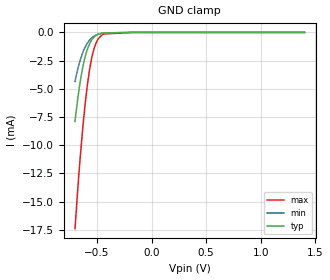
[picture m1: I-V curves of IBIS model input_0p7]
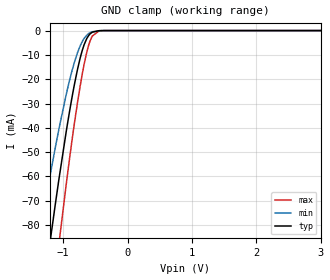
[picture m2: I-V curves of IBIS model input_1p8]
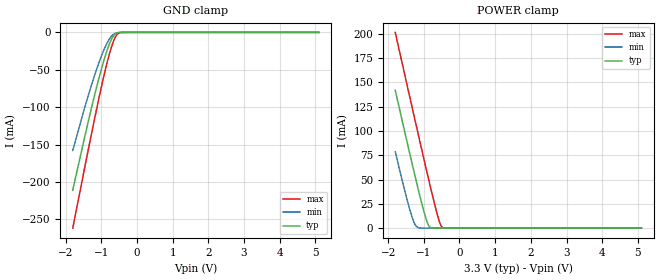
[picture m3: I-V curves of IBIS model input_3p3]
| Texas Instruments Incorporated
| SN74AXC4T774 4-Bit Dual-Supply Bus Transceiver with Independent Direction
| Control, Configurable Voltage Translation, and Tri-State Outputs
[IBIS Ver]   4.1
[File name]   sn74axc4t774.ibs
[Date]   04/15/2019
[File Rev]   1.0
[Source]
| Texas Instruments Incorporated.
| Analog-eLab Design Center, HPA
| 12500 TI Blvd
| Dallas, TX -75243
[Notes]   Revision History:
| Rev 1.0: 04/15/2019
| - Initial version of the model
| - Model generated from simulations in SPECTRE
| - C_comp although listed in numerical order of value are
|   obtained from varying PVT conditions. For PVT conditions for
|   each specific value refer the buffer description under
|   respective [Model]. IBIS model user is responsible for using
|   appropriate C_comp to simulate for Signal Integrity.
| - Warnings regarding combined Non-monotonicity of various models have been
|   reviewd and considered minor and can be ignored.
| - Model names with a trailing _0p7 contain the model for 0.7V operation.
|   Model names with a trailing _1p8 contain the model for 1.8V operation.
|   Model names with a trailing _3p3 contain the model for 3.3V operation.
[Disclaimer]
| This model is designed as an aid for customers of Texas Instruments.
| TI and its licensors and suppliers make no warranties, either expressed
| or implied, with respect to this  model, including the warranties of
| merchantability or fitness for a particular purpose. The model is
| provided solely on an "as is" basis. The entire risk as to its quality
| and performance is with the customer.
| This model is subject to change without notice. Texas Instruments
| Incorporated is not responsible for updating this model.
[Copyright]
(C) Copyright 2019 Texas Instruments Incorporated.All rights reserved.
|  Component SN74AXC4T774BQB 16-Pin VQFN - BQB package
|  Part # SN74AXC4T774BQB
[Component]   SN74AXC4T774BQB
[Manufacturer]  TI
[Package]   |16 VQFN - BQB package
|   typ   min   max
R_pkg   0.05   0.04   0.06
L_pkg   1.0nH   0.8nH   1.2nH
C_pkg   0.2pF   0.16pF   0.24pF
[Pin]  signal_name model_name   R_pin   L_pin   C_pin
1   DIR1   input   NA   NA   NA
2   DIR2   input   NA   NA   NA
3   A1   io   NA   NA   NA
4   A2   io   NA   NA   NA
5   A3   io   NA   NA   NA
6   A4   io   NA   NA   NA
7   DIR3   input   NA   NA   NA
8   DIR4   input   NA   NA   NA
9   nOE   input   NA   NA   NA
10   GND   gnd   NA   NA   NA
11   B4   io   NA   NA   NA
12   B3   io   NA   NA   NA
13   B2   io   NA   NA   NA
14   B1   io   NA   NA   NA
15   VCCB   power   NA   NA   NA
16   VCCA   power   NA   NA   NA
|  Component SN74AXC4T774PW 16-Pin TSSOP - PW package
|  Part # SN74AXC4T774PW
[Component]   SN74AXC4T774PW
[Manufacturer]  TI
[Package]   |16 TSSOP - PW package
|   typ   min   max
R_pkg   0.05   0.04   0.06
L_pkg   1.0nH   0.8nH   1.2nH
C_pkg   0.2pF   0.16pF   0.24pF
[Pin]  signal_name model_name   R_pin   L_pin   C_pin
1   DIR1   input   NA   NA   NA
2   DIR2   input   NA   NA   NA
3   A1   io   NA   NA   NA
4   A2   io   NA   NA   NA
5   A3   io   NA   NA   NA
6   A4   io   NA   NA   NA
7   DIR3   input   NA   NA   NA
8   DIR4   input   NA   NA   NA
9   nOE   input   NA   NA   NA
10   GND   gnd   NA   NA   NA
11   B4   io   NA   NA   NA
12   B3   io   NA   NA   NA
13   B2   io   NA   NA   NA
14   B1   io   NA   NA   NA
15   VCCB   power   NA   NA   NA
16   VCCA   power   NA   NA   NA
|  Component SN74AXC4T774RSV 16-Pin UQFN - RSV package
|  Part # SN74AXC4T774RSV
[Component]   SN74AXC4T774RSV
[Manufacturer]  TI
[Package]   |16 UQFN - RSV package
|   typ   min   max
R_pkg   0.05   0.04   0.06
L_pkg   1.0nH   0.8nH   1.2nH
C_pkg   0.2pF   0.16pF   0.24pF
[Pin]  signal_name model_name   R_pin   L_pin   C_pin
1   A1   io   NA   NA   NA
2   A2   io   NA   NA   NA
3   A3   io   NA   NA   NA
4   A4   io   NA   NA   NA
5   DIR3   input   NA   NA   NA
6   DIR4   input   NA   NA   NA
7   nOE   input   NA   NA   NA
8   GND   gnd   NA   NA   NA
9   B4   io   NA   NA   NA
10   B3   io   NA   NA   NA
11   B2   io   NA   NA   NA
12   B1   io   NA   NA   NA
13   VCCB   power   NA   NA   NA
14   VCCA   power   NA   NA   NA
15   DIR1   input   NA   NA   NA
16   DIR2   input   NA   NA   NA
|   Model Selectors
[Model Selector] input
input_0p7   0.7V   digital Input
input_1p8   1.8V   digital Input
input_3p3   3.3V   digital Input
[Model Selector] io
io_0p7_x   0.7V   digital I/O   |Output = 0.7V; Input = 3.3V
io_0p7_y   0.7V   digital I/O   |Output = 0.7V; Input = 1.8V
io_0p7_z   0.7V   digital I/O   |Output = 0.7V; Input = 0.7V
io_1p8_x   1.8V   digital I/O   |Output = 1.8V; Input = 3.3V
io_1p8_y   1.8V   digital I/O   |Output = 1.8V; Input = 1.8V
io_1p8_z   1.8V   digital I/O   |Output = 1.8V; Input = 0.7V
io_3p3_x   3.3V   digital I/O   |Output = 3.3V; Input = 3.3V
io_3p3_y   3.3V   digital I/O   |Output = 3.3V; Input = 1.8V
io_3p3_z   3.3V   digital I/O   |Output = 3.3V; Input = 0.7V
| Models and submodels in the file (12): input_0p7 (Input), input_1p8 (Input), input_3p3 (Input), io_0p7_x (I/O), io_0p7_y (I/O), io_0p7_z (I/O), io_1p8_x (I/O), io_1p8_y (I/O), io_1p8_z (I/O), io_3p3_x (I/O), io_3p3_y (I/O), io_3p3_z (I/O)
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|   input_0p7 Model
[Model]   input_0p7
Model_type   Input
Vinl = 0.21
Vinh = 0.49
|   typ   min   max
C_comp   0.744pF   0.651pF   0.903pF
[Model spec]
|subparameter
Vinl   0.21   0.195   0.225
Vinh   0.49   0.455   0.525
| Where Nom  PVT is Nominal Process, 0.7V, 27C
|   Fast PVT is Strong Process,  0.75V, -40C
|   Slow PVT is Weak Process,   0.65V, 130C
[Voltage Range]   0.7   0.65   0.75
|Junction Temperature
[Temperature Range]   27   130   -40
[Power Clamp Reference]   0.7   0.65   0.75
[GND Clamp Reference]   0   0   0
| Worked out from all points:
|   GND clamp passes 1 mA (typ) near -0.57 V on its own axis
[GND Clamp]
|   Voltage   I(typ)   I(min)   I(max)
-700mV    -7.896mA   -4.354mA   -17.4mA
-676.9mV  -6.033mA   -3.335mA   -14.2mA
-651.7mV  -4.329mA   -2.43mA    -11.02mA
-624.4mV  -2.873mA   -1.673mA   -7.992mA
-588.7mV  -1.545mA   -978.4uA   -4.797mA
-567.7mV  -1.026mA   -696.2uA   -3.358mA
-548.8mV  -691.6uA   -504.6uA   -2.342mA
-527.8mV  -434.7uA   -346.8uA   -1.503mA
-487.9mV  -168.3uA   -161.7uA   -574.9uA
-454.3mV  -71.1uA    -80.61uA   -230.7uA
-175mV    -4.812nA   -77.92nA   0A
1.4V      0A         0A         0A
[POWER Clamp]
|   Voltage   I(typ)   I(min)   I(max)
-700mV    0A         0A         0A
0V        0A         0A         0A
1.4V      0A         0A         0A
|   input_1p8 Model
[Model]   input_1p8
Model_type   Input
Vinl = 0.63
Vinh = 1.17
|   typ   min   max
C_comp   1.405pF   0.843pF   2.003pF
[Model spec]
|subparameter
Vinl   0.63   0.567   0.693
Vinh   1.17   1.053   1.287
| Where Nom  PVT is Nominal Process, 1.8V, 27C
|   Fast PVT is Strong Process,  1.98V, -40C
|   Slow PVT is Weak Process,   1.62V, 130C
[Voltage Range]   1.8   1.62   1.98
|Junction Temperature
[Temperature Range]   27   130   -40
[Power Clamp Reference]   1.8   1.62   1.98
[GND Clamp Reference]   0   0   0
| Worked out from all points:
|   GND clamp passes 1 mA (typ) near -0.56 V on its own axis
[GND Clamp]
|   Voltage   I(typ)   I(min)   I(max)
-1.8V     -210.9mA   -157.9mA   -261.6mA
-1.319V   -109.8mA   -77.26mA   -146mA
-1.206V   -87.46mA   -60.12mA   -119.6mA
-1.12V    -71.04mA   -47.78mA   -99.81mA
-1.066V   -61.14mA   -40.45mA   -87.72mA
-952.2mV  -41.52mA   -26.26mA   -63.25mA
-903.6mV  -33.72mA   -20.8mA    -53.27mA
-779.4mV  -16.26mA   -9.28mA    -30.01mA
-676.8mV  -6.025mA   -3.331mA   -14.19mA
-579.6mV  -1.299mA   -846.1uA   -4.132mA
-385.2mV  -10.15uA   -16.94uA   -26.1uA
3.6V      0A         0A         0A
[POWER Clamp]
|   Voltage   I(typ)   I(min)   I(max)
-1.8V     0A         0A         0A
0V        0A         0A         0A
3.6V      0A         0A         0A
|   input_3p3 Model
[Model]   input_3p3
Model_type   Input
Vinl = 0.8
Vinh = 2
|   typ   min   max
C_comp   1.869pF   1.275pF   2.146pF
| Where Nom  PVT is Nominal Process, 3.3V, 27C
|   Fast PVT is Strong Process,  3.6V, -40C
|   Slow PVT is Weak Process,   3.0V, 130C
[Voltage Range]   3.3   3   3.6
|Junction Temperature
[Temperature Range]   27   130   -40
[Power Clamp Reference]   3.3   3   3.6
[GND Clamp Reference]   0   0   0
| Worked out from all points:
|   GND clamp passes 1 mA (typ) near -0.57 V on its own axis
|   POWER clamp passes 1 mA (typ) near -0.83 V on its own axis
[GND Clamp]
|   Voltage   I(typ)   I(min)   I(max)
-1.8V     -210.9mA   -157.9mA   -261.6mA
-1.49V    -144.7mA   -104.6mA   -186.5mA
-1.296V   -105.2mA   -73.69mA   -140.6mA
-1.117V   -70.54mA   -47.4mA    -99.2mA
-951.3mV  -41.37mA   -26.15mA   -63.06mA
-820.2mV  -21.52mA   -12.61mA   -37.23mA
-716.7mV  -9.415mA   -5.207mA   -19.86mA
-613.2mV  -2.39mA    -1.422mA   -6.892mA
-523.5mV  -394uA     -320.5uA   -1.365mA
-426.9mV  -33.77uA   -44.19uA   -102.3uA
-68.1mV   0A         0A         0A
5.1V      0A         0A         0A
[POWER Clamp]
|   Voltage   I(typ)   I(min)   I(max)
-1.8V     141.9mA    78.74mA    201.4mA
-1.414V   79.93mA    21.78mA    138.3mA
-1.296V   61.5mA     8.016mA    119.2mA
-1.234V   51.89mA    3.123mA    109.2mA
-1.151V   39.29mA    456.6uA    95.81mA
-985.8mV  15.65mA    4.19uA     69.3mA
-868.5mV  3.093mA    132.8nA    50.79mA
-799.5mV  400.9uA    8.626nA    40.08mA
-571.8mV  48.29nA    0A         7.669mA
-516.6mV  0A         0A         2.383mA
-468.3mV  0A         0A         390.4uA
5.1V      0A         0A         0A
